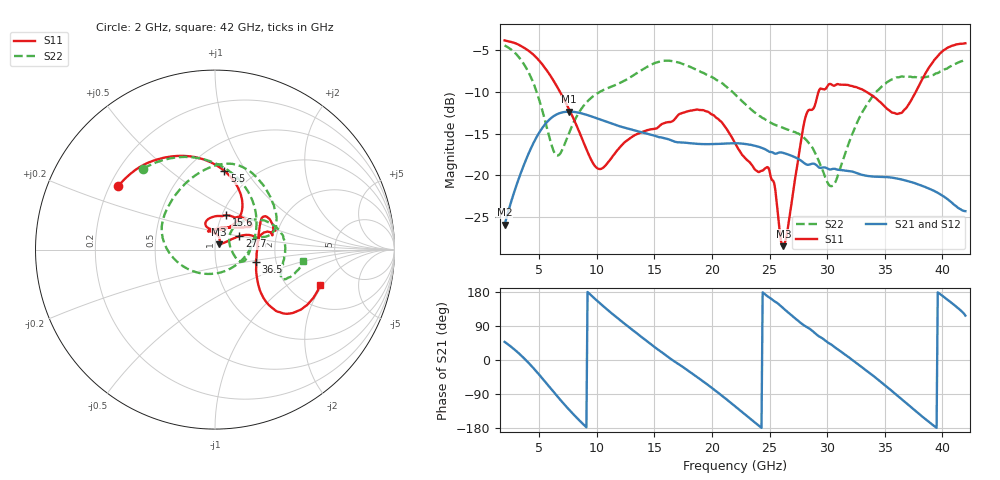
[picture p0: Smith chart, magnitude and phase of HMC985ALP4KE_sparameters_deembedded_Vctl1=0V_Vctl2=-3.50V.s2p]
!s2p File: Measurements: S11, S21, S12, S22
# GHz S dB R 50.0
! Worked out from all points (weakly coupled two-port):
!   401 points, 2 GHz to 42 GHz, reference 50 ohm
!   highest |S21| = -12.37 dB at 7.6 GHz (marker M1); lowest = -26.0 dB at 2 GHz (marker M2)
!   lowest |S11| = -28.5 dB at 26.2 GHz (marker M3), VSWR 1.08, Z = 52.3 + j3.07 ohm
!   |S11| at or under -10 dB: 6.811 GHz to 29.25 GHz (22.44 GHz wide, 124 % of centre); 33.41 GHz to 37.69 GHz (4.279 GHz wide, 12 % of centre)
!   |S22| runs from -21.3 to -4.4 dB; largest |S21 - S12| = 0.00037
!   S11 on the Smith chart (normalised r, x): 2 GHz: 0.23, +0.28; 5.5 GHz: 0.74, +0.80; 15.6 GHz: 1.05, +0.42; 27.7 GHz: 1.30, +0.20; 36.5 GHz: 1.57, -0.23; 42 GHz: 2.94, -1.89
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2  -3.81 146.7  -25.97 47.8  -25.96 47.9  -4.41 131.5
3.6  -4.62 119.7  -19.04 7.2  -19.05 7.2  -6.51 87.4
5.5  -7.11 83.2  -13.91 -56.7  -13.91 -56.7  -13.39 9.8
6.5  -9.24 65.9  -12.72 -93.1  -12.71 -93.1  -17.61 -66.1
7.6  -12.09 54.0  -12.37 -131.2  -12.37 -131.2  -14.91 -140.8
8.7  -15.54 54.5  -12.59 -165.8  -12.59 -165.8  -11.96 -174.9
10.3  -19.27 88.4  -13.32 149.0  -13.30 149.0  -9.97 159.3
12.6  -15.86 109.1  -14.38 91.2  -14.38 91.2  -8.50 125.8
15.4  -14.16 75.4  -15.44 25.9  -15.45 25.8  -6.37 84.2
15.6  -13.91 71.8  -15.47 21.4  -15.48 21.4  -6.31 81.8
19.3  -12.22 33.5  -16.28 -57.9  -16.28 -57.9  -7.74 36.9
22  -16.13 51.5  -16.18 -122.0  -16.17 -122.0  -10.29 14.5
24.9  -19.11 104.4  -17.14 166.4  -17.13 166.4  -13.54 11.5
26.2  -28.55 51.7  -17.33 136.3  -17.33 136.2  -14.33 -4.1
27.7  -16.17 28.8  -18.24 97.9  -18.25 97.9  -15.19 -21.6
28.7  -12.14 12.7  -18.63 77.3  -18.62 77.2  -16.67 -24.9
30.5  -9.22 18.3  -19.25 37.7  -19.25 37.7  -21.27 19.9
33  -9.67 34.1  -19.96 -18.9  -19.95 -18.9  -12.56 43.5
35.4  -12.23 11.7  -20.27 -76.2  -20.27 -76.2  -8.68 18.5
36.5  -12.48 -16.6  -20.54 -104.4  -20.54 -104.4  -8.15 6.2
39.5  -5.86 -43.6  -22.06 -179.0  -22.05 -179.0  -7.76 -23.2
42  -4.15 -18.6  -24.34 117.1  -24.36 117.1  -6.16 -7.1
